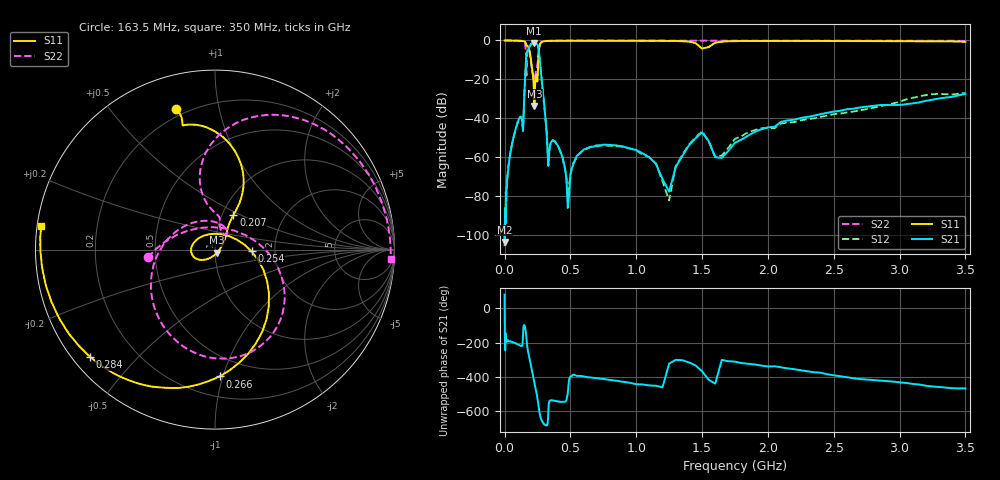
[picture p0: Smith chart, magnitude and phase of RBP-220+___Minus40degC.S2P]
! Mini-Circuits
! S2P DATA File Format
! Type: BAND PASS FILTER
! Model: RBP-220+
! All S Parameters are in dB deg format
! TEST CONDITIONS: INPUT POWER = 0 dBm @ Temperature = - 40 deg C
! 401 Frequency points
# MHz S DB R 50
!FREQ  MAG(S11)PHS(S11)MAG(S21)PHS(S21)MAG(S12)PHS(S12)MAG(S22)PHS(S22)
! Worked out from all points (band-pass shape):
!   401 points, 500 kHz to 3.5 GHz, reference 50 ohm
!   highest |S21| = -1.39 dB at 222 MHz (marker M1); lowest = -103.7 dB at 500 kHz (marker M2)
!   |S21| within 3 dB of the highest: 183.5 MHz to 258.4 MHz (74.93 MHz wide, 33.9 % of centre)
!   lowest |S11| = -33.7 dB at 227 MHz (marker M3), VSWR 1.04, Z = 51 - j1.82 ohm
!   |S11| at or under -10 dB: 200.7 MHz to 256.5 MHz (55.84 MHz wide, 24.4 % of centre)
!   |S22| runs from -20.0 to 0.0 dB; largest |S21 - S12| = 0.012
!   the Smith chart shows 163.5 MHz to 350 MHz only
!   S11 on the Smith chart (normalised r, x): 163.5 MHz: 0.16, +0.75; 207 MHz: 1.13, +0.46; 254 MHz: 1.51, -0.03; 266 MHz: 0.35, -0.98; 284 MHz: 0.05, -0.37; 350 MHz: 0.01, +0.07
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0.5  -0.02 179.9  -103.73 80.0  -105.83 177.3  -0.01 -0.1
2.5  -0.02 179.3  -101.78 -165.9  -95.98 152.6  0.00 -0.9
10  -0.03 177.5  -77.83 164.3  -83.50 -162.2  -0.01 -3.5
42.5  -0.07 169.3  -58.46 167.6  -58.51 166.5  0.00 -13.9
140  -0.31 131.4  -46.52 -168.2  -46.50 -167.1  -0.33 -72.6
163.5  -1.78 105.4  -9.55 -153.9  -9.49 -154.4  -8.48 -173.3
183  -3.71 89.2  -4.46 91.3  -4.49 91.1  -4.42 -93.6
207  -13.23 61.9  -1.60 -0.8  -1.60 -1.1  -14.65 122.8
222  -24.20 40.0  -1.39 -54.5  -1.39 -54.5  -19.18 53.0
227  -33.70 -59.8  -1.42 -72.3  -1.41 -72.4  -20.02 61.4
254  -13.80 -2.7  -2.93 173.0  -2.97 172.8  -9.20 103.1
266  -3.01 -87.9  -8.82 109.0  -8.90 110.2  -2.36 74.8
284  -0.75 -139.3  -21.62 61.9  -21.53 61.9  -0.65 38.9
330  -0.24 -179.3  -62.54 71.0  -62.03 74.0  -0.22 5.2
350  -0.21 172.3  -52.85 -177.3  -52.84 -176.5  -0.17 -3.1
480  -0.15 142.2  -86.21 -136.1  -79.96 -146.6  -0.08 -35.8
850  -0.13 89.2  -54.01 -63.2  -54.39 -67.2  -0.07 -92.8
1200  -0.18 39.8  -71.30 -101.6  -72.66 -90.7  -0.07 -138.3
1550  -3.39 118.2  -51.71 -57.3  -51.74 -58.2  -0.12 177.7
1800  -0.26 0.5  -50.99 40.0  -49.21 35.9  -0.14 148.0
2300  -0.26 -71.9  -39.33 -8.1  -40.51 -14.7  -0.13 90.8
3500  -0.64 138.5  -27.46 -108.5  -27.00 -118.7  -0.26 -57.5
